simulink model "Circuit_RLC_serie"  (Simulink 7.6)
settings: Solver=ode23t  StartTime=0.0  StopTime=0.04  RelTol=1e-3
InitFcn:
  | clc
  | clear all
  | delete *.mat
StopFcn:
  | close all
  | load Circuit_RLC.mat
  | plot(x(1,:),x(2,:),x(1,:),x(3,:),x(1,:),x(4,:))
  | grid
  | title('Courant et tension - circuit RLC série')
  | xlabel('temps')
libraries: powerlib x9

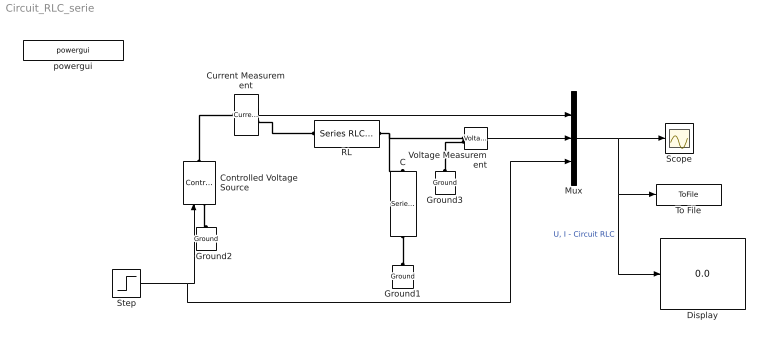
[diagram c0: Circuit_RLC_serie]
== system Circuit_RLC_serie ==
  C : powerlib/Elements/Series RLC Branch  DialogController=POWERSYS.PowerSysDialog  PhysicalDomain=powersysdomain  SubClassName=unknown  LeftPortType=p1  RightPortType=p1  LConnTagsString=__new0  RConnTagsString=__new0  BranchType=C  Resistance=1  Inductance=1e-3  SetiL0=off  InitialCurrent=0  Capacitance=0.001  Setx0=off  InitialVoltage=0  Measurements=None
  Controlled Voltage Source : powerlib/Electrical Sources/Controlled Voltage Source  DialogController=POWERSYS.PowerSysDialog  SystemSampleTime=-1  Initialize=on  Source_Type=AC  Amplitude=0  Phase=0  Frequency=0  Measurements=None
  Current Measurement : powerlib/Measurements/Current Measurement  DialogController=POWERSYS.PowerSysDialog  SystemSampleTime=-1  PhasorSimulation=off  OutputType=Complex  PSBequivalent=0
  Display : Display
  Ground1 : powerlib/Elements/Ground  DialogController=POWERSYS.PowerSysDialog  PhysicalDomain=powersysdomain  SubClassName=unknown  LeftPortType=p1  RightPortType=p1  LConnTagsString=a
  Ground2 : powerlib/Elements/Ground  DialogController=POWERSYS.PowerSysDialog  PhysicalDomain=powersysdomain  SubClassName=unknown  LeftPortType=p1  RightPortType=p1  LConnTagsString=a
  Ground3 : powerlib/Elements/Ground  DialogController=POWERSYS.PowerSysDialog  PhysicalDomain=powersysdomain  SubClassName=unknown  LeftPortType=p1  RightPortType=p1  LConnTagsString=a
  Mux : Mux  Inputs=3
  RL : powerlib/Elements/Series RLC Branch  DialogController=POWERSYS.PowerSysDialog  PhysicalDomain=powersysdomain  SubClassName=unknown  LeftPortType=p1  RightPortType=p1  LConnTagsString=__new0  RConnTagsString=__new0  BranchType=RL  Resistance=4  Inductance=10e-3  SetiL0=off  InitialCurrent=0  Capacitance=0  Setx0=off  InitialVoltage=0  Measurements=None
  Scope : Scope
  Step : Step  Time=0  SampleTime=0
  To File : ToFile  Filename=Circuit_RLC  MatrixName=x
  Voltage Measurement : powerlib/Measurements/Voltage Measurement  DialogController=POWERSYS.PowerSysDialog  SystemSampleTime=-1  PhasorSimulation=off  OutputType=Complex  PSBequivalent=0
  powergui : powerlib/powergui  Priority=1  SystemSampleTime=-1  SimulationMode=Continuous  SampleTime=50e-6  frequency=60  SPID=off  DisableSnubberDevices=off  DisableRonSwitches=off  DisableVfSwitches=off  SwTol=0  Interpol=off  frequencyindice=0  echomessages=off  HookPort=off  DisplayEquations=off  FunctionMessages=off  EnableUseOfTLC=off  x0status=blocks  RestoreLinks=warning  ResistiveCurrentMeasurement=off  Ylog=off  Xlog=on  ShowGrid=off  save=off  variable=ZData  ZoomFFT=off  StartTime=0.0  cycles=1  DisplayStyle=1  fundamental=60  FreqAxis=off  MaxFrequency=1000  frequencyindicesteady=1  display=off  methode=off
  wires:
  Voltage Measurement/1 -> Mux/2
  Current Measurement/1 -> Mux/1
  Step/1 -> Controlled Voltage Source/1, Mux/3
  Mux/1 -> Scope/1, To File/1, Display/1  "U, I - Circuit RLC"
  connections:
  Current Measurement/RConn1 -- RL/LConn1
  RL/RConn1 -- C/LConn1 -- Voltage Measurement/LConn1
  C/RConn1 -- Ground1/LConn1
  Controlled Voltage Source/RConn1 -- Current Measurement/LConn1
  Controlled Voltage Source/LConn1 -- Ground2/LConn1
  Ground3/LConn1 -- Voltage Measurement/LConn2
